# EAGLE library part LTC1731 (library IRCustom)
Linear Tech LTC1731 lipoly charger By microbuilder.eu
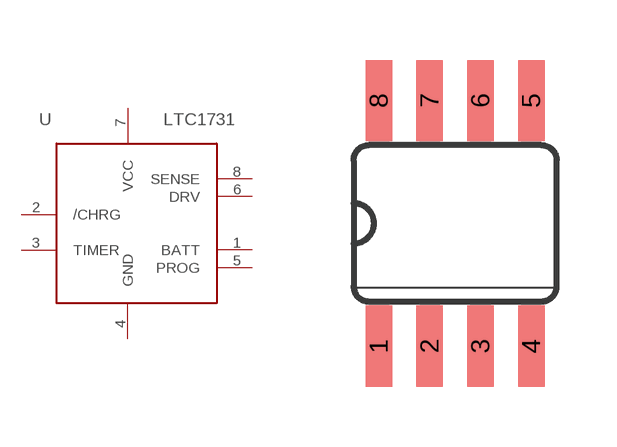
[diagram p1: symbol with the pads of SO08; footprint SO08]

Designator prefix -

## LTC1731  [SO08]
1  BATT  out
2  /CHRG
3  TIMER  pas
4  GND  sup
5  PROG  pas
6  DRV  out
7  VCC  sup
8  SENSE

## Footprint SO08 (pad centres in mm)
smd 0.66 x 2.032: 1 -1.905,-3.073; 2 -0.635,-3.073; 3 0.635,-3.073; 4 1.905,-3.073; 5 1.905,3.073; 6 0.635,3.073; 7 -0.635,3.073; 8 -1.905,3.073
